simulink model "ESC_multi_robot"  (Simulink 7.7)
settings: Solver=ode3  StartTime=starttime  StopTime=stoptime  FixedStep=stepsize  RelTol=1e-3
PreLoadFcn:
  | load ESC_GUI_params_multi
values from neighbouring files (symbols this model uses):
  Kd = 60    [sim_run_multi.m]    (also in sim_run_uni.m)
  Kp = 3000    [sim_run_multi.m]    (also in sim_run_uni.m)
  noise_max = value    [ESC_GUI_multi.m]    (also in ESC_GUI_uni.m; sim_run_multi.m = 0.01; sim_run_uni.m = 0.2)
  switch_noise = 1    [ESC_GUI_multi.m]    (also in ESC_GUI_uni.m; sim_run_multi.m; sim_run_uni.m)
  switch_optimizer = method_no+1    [ESC_GUI_multi.m]    (also in ESC_GUI_uni.m = method_no; sim_run_multi.m = 4; sim_run_uni.m = 1)
  x0 = [0;0]    [sim_run_multi.m]    (also in sim_run_uni.m = 0)
undefined symbols (not defined in the file or in its folder): approx, nn, perturb
libraries: roblocks x8, simulink x1, commnoisgen2 x1

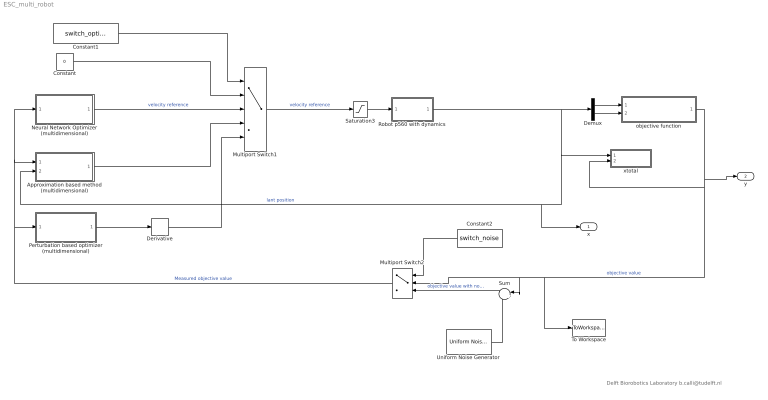
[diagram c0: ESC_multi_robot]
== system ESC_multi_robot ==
  note: Delft Biorobotics Laboratory b.calli@tudelft.nl
  Approximation based method (multidimensional) : Subsystem  mask{K_grad=approx.K_grad, sampling=approx.sampling, data_size=approx.data_size, vel_init=approx.vel_init, lpf_constant=approx.filter_constant}
      mask prompts: K_grad "Gain"; data_size "Data size"; vel_init "Initial velocity"; lpf_constant "Low pass filter constant"
  Constant : Constant  Value=0
  Constant1 : Constant  Value=switch_optimizer
  Constant2 : Constant  Value=switch_noise
  Demux : Demux  Outputs=2
  Derivative : Derivative
  Multiport Switch1 : MultiPortSwitch  Inputs=4  zeroidx=off
  Multiport Switch2 : MultiPortSwitch  Inputs=2  zeroidx=off
  Neural Network Optimizer (multidimensional) : Subsystem  mask{M=nn.M, A=nn.A, B=nn.B, ddelta1=nn.ddelta1, ddelta2=nn.ddelta2, ddelta3=nn.ddelta3, delta=nn.delta, mpd_init=nn.mpd_init}
      mask prompts: ddelta1 "Direction 1 delta"; ddelta2 "Direction 2 delta"; ddelta3 "Direction 3 delta"; mpd_init "Minimum Peak Detector initial value"
  Perturbation based optimizer (multidimensional) : Subsystem  mask{corr_gain=perturb.corr_gain, low_pass_pole=perturb.low_pass_pole, high_pass_pole=perturb.high_pass_pole, sine_amp=perturb.sine_amp, sine_freq=perturb.sine_freq, sine_phase=perturb.sine_phase, comp_zero=perturb.comp_zero, comp_pole=perturb.comp_pole}
      mask prompts: corr_gain "Correction gain"; low_pass_pole "Low Pass Filter pole"; high_pass_pole "High Pass Filter pole"; sine_amp "Sinus amplitude"; sine_freq "Sinus frequency"; sine_phase "Sinus phase"; comp_zero "Compensator zero"; comp_pole "Compensator pole"
  Robot p560 with dynamics : Subsystem
  Saturation3 : Saturate  UpperLimit=1  LowerLimit=-1
  Sum : Sum  Inputs=|++
  To Workspace : ToWorkspace  VariableName=y  SampleTime=-1  SaveFormat=Structure With Time
  Uniform Noise Generator : commnoisgen2/Uniform Noise Generator  SystemSampleTime=-1  low=-noise_max  up=noise_max  seed=31  Ts=0.001  frameBased=off  sampPerFrame=1  orient=off  outDataType=double
  objective function : Stateflow chart  TreatAsAtomicUnit=on
  xtotal : Subsystem
  x : Outport
  y : Outport  Port=2
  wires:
  Robot p560 with dynamics/1(x) -> xtotal/1(x), Approximation based method (multidimensional)/2(x), x/1, Demux/1  "lant position"
  Neural Network Optimizer (multidimensional)/1(xdot_ref) -> Multiport Switch1/3  "velocity reference"
  Constant/1 -> Multiport Switch1/2
  Constant1/1 -> Multiport Switch1/1
  objective function/1(y) -> Multiport Switch2/2, Sum/1, To Workspace/1, xtotal/2(y), y/1  "objective value"
  Uniform Noise Generator/1 -> Sum/2
  Sum/1 -> Multiport Switch2/3  "objective value with noise"
  Constant2/1 -> Multiport Switch2/1
  Approximation based method (multidimensional)/1(xdot_ref) -> Multiport Switch1/4
  Multiport Switch1/1 -> Saturation3/1  "velocity reference"
  Demux/1 -> objective function/1(x1)
  Perturbation based optimizer (multidimensional)/1(xref) -> Derivative/1
  Derivative/1 -> Multiport Switch1/5
  Multiport Switch2/1 -> Approximation based method (multidimensional)/1(y), Neural Network Optimizer (multidimensional)/1(y), Perturbation based optimizer (multidimensional)/1(y)  "Measured objective value"
  Demux/2 -> objective function/2(x2)
  Saturation3/1 -> Robot p560 with dynamics/1(xref)

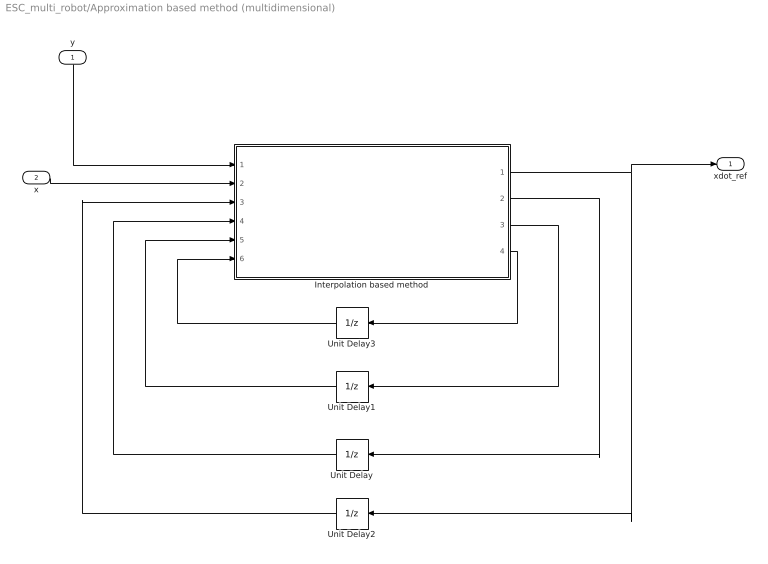
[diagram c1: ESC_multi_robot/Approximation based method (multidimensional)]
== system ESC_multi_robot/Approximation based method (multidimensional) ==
  y : Inport
  x : Inport  Port=2
  Interpolation based method : Stateflow chart  TreatAsAtomicUnit=on
  Unit Delay : UnitDelay  X0=[zeros(1,data_size);zeros(1,data_size)]  SampleTime=-1
  Unit Delay1 : UnitDelay  X0=zeros(1,data_size)  SampleTime=-1
  Unit Delay2 : UnitDelay  X0=[0;0]  SampleTime=-1
  Unit Delay3 : UnitDelay  SampleTime=-1
  xdot_ref : Outport
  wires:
  Unit Delay/1 -> Interpolation based method/4(x_data)
  Unit Delay1/1 -> Interpolation based method/5(y_data)
  y/1 -> Interpolation based method/1(y_data_in)
  x/1 -> Interpolation based method/2(x_data_in)
  Unit Delay2/1 -> Interpolation based method/3(xdot_ref_in)
  Unit Delay3/1 -> Interpolation based method/6(sample)
  Interpolation based method/4(sample_out) -> Unit Delay3/1
  Interpolation based method/3(y_data_out) -> Unit Delay1/1
  Interpolation based method/2(x_data_out) -> Unit Delay/1
  Interpolation based method/1(xdot_ref) -> Unit Delay2/1, xdot_ref/1

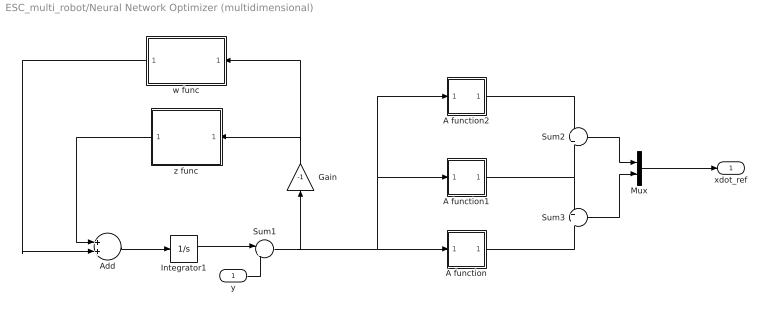
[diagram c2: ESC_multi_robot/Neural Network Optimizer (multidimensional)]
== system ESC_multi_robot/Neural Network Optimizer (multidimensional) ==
  y : Inport
  A function : Subsystem
  A function1 : Subsystem
  A function2 : Subsystem
  Add : Sum
  Gain : Gain  Gain=-1
  Integrator1 : Integrator  InitialCondition=mpd_init
  Mux : Mux  Inputs=2
  Sum1 : Sum  Inputs=|+-
  Sum2 : Sum  Inputs=+|+
  Sum3 : Sum  Inputs=+|+
  w func : Subsystem
  z func : Subsystem
  xdot_ref : Outport
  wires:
  Sum1/1 -> Gain/1, A function/1(e), A function1/1(e), A function2/1(e)
  Gain/1 -> w func/1(e_minus), z func/1(e_minus)
  w func/1(w) -> Add/2
  z func/1(z) -> Add/1
  Add/1 -> Integrator1/1
  Integrator1/1 -> Sum1/1
  A function2/1(xdot) -> Sum2/1
  A function1/1(xdot) -> Sum2/2, Sum3/1
  A function/1(xdot) -> Sum3/2
  Sum2/1 -> Mux/1
  Sum3/1 -> Mux/2
  Mux/1 -> xdot_ref/1
  y/1 -> Sum1/2

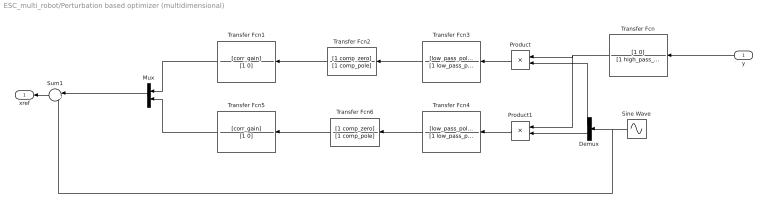
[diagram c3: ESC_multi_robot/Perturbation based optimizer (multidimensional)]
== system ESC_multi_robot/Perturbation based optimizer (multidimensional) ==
  y : Inport
  Demux : Demux  Outputs=2
  Mux : Mux  Inputs=2
  Product : Product  Multiplication=Matrix(*)
  Product1 : Product  Multiplication=Matrix(*)
  Sine Wave : Sin  Amplitude=[sine_amp sine_amp]  Frequency=[sine_freq sine_freq]  Phase=[0 sine_phase]  SampleTime=0
  Sum1 : Sum  Inputs=|++
  Transfer Fcn : TransferFcn  Numerator=[1 0]  Denominator=[1 high_pass_pole]
  Transfer Fcn1 : TransferFcn  Numerator=[corr_gain]  Denominator=[1 0]
  Transfer Fcn2 : TransferFcn  Numerator=[1 comp_zero]  Denominator=[1 comp_pole]
  Transfer Fcn3 : TransferFcn  Numerator=[low_pass_pole]  Denominator=[1 low_pass_pole]
  Transfer Fcn4 : TransferFcn  Numerator=[low_pass_pole]  Denominator=[1 low_pass_pole]
  Transfer Fcn5 : TransferFcn  Numerator=[corr_gain]  Denominator=[1 0]
  Transfer Fcn6 : TransferFcn  Numerator=[1 comp_zero]  Denominator=[1 comp_pole]
  xref : Outport
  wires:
  y/1 -> Transfer Fcn/1
  Sum1/1 -> xref/1
  Transfer Fcn/1 -> Product/1, Product1/1
  Sine Wave/1 -> Demux/1, Sum1/2
  Demux/1 -> Product/2
  Demux/2 -> Product1/2
  Product/1 -> Transfer Fcn3/1
  Product1/1 -> Transfer Fcn4/1
  Transfer Fcn3/1 -> Transfer Fcn2/1
  Transfer Fcn4/1 -> Transfer Fcn6/1
  Transfer Fcn1/1 -> Mux/1
  Transfer Fcn5/1 -> Mux/2
  Mux/1 -> Sum1/1
  Transfer Fcn2/1 -> Transfer Fcn1/1
  Transfer Fcn6/1 -> Transfer Fcn5/1

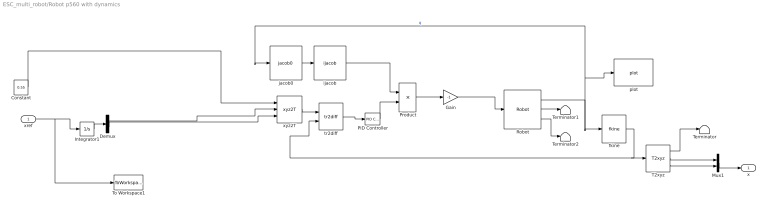
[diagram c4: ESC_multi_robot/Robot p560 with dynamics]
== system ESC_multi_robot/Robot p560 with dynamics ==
  xref : Inport
  Constant : Constant  Value=0.55
  Demux : Demux  Outputs=2
  Gain : Gain  Gain=-1
  Integrator1 : Integrator  InitialCondition=x0
  Mux1 : Mux  Inputs=2
  PID Controller : simulink/Continuous/PID Controller  SystemSampleTime=-1  Controller=PID  TimeDomain=Continuous-time  SampleTime=1  IntegratorMethod=Forward Euler  FilterMethod=Forward Euler  Form=Parallel  P=[Kp Kp Kp Kp Kp Kp]  I=[0 0 0 0 0 0]  D=[Kd Kd Kd Kd Kd Kd]  N=100  InitialConditionSource=internal  InitialConditionForIntegrator=0  InitialConditionForFilter=0  ExternalReset=none  LimitOutput=off  UpperSaturationLimit=inf  LowerSaturationLimit=-inf  LinearizeAsGain=off  AntiWindupMode=none  Kb=1  TrackingMode=off  Kt=1  PParamMin=[]  PParamMax=[]  IParamMin=[]  IParamMax=[]  DParamMin=[]  DParamMax=[]  NParamMin=[]  NParamMax=[]  KbParamMin=[]  KbParamMax=[]  KtParamMin=[]  KtParamMax=[]  POutMin=[]  POutMax=[]  IOutMin=[]  IOutMax=[]  DOutMin=[]  DOutMax=[]  NOutMin=[]  NOutMax=[]  KbOutMin=[]  KbOutMax=[]  KtOutMin=[]  KtOutMax=[]  IntegratorOutMin=[]  IntegratorOutMax=[]  FilterOutMin=[]  FilterOutMax=[]  SumOutMin=[]  SumOutMax=[]  SumI1OutMin=[]  SumI1OutMax=[]  SumI2OutMin=[]  SumI2OutMax=[]  SumI3OutMin=[]  SumI3OutMax=[]  SumDOutMin=[]  SumDOutMax=[]  SaturationOutMin=[]  SaturationOutMax=[]  IntegratorContinuousStateAttributes=''  IntegratorStateMustResolveToSignalObject=off  IntegratorRTWStateStorageClass=Auto  FilterContinuousStateAttributes=''  FilterStateMustResolveToSignalObject=off  FilterRTWStateStorageClass=Auto
  Product : Product  Multiplication=Matrix(*)
  Robot : roblocks/Robot  SystemSampleTime=-1  robot=p560  q0="[0.2763    0.9125    2.9359         0    2.4348   -0.2763]"
  T2xyz : roblocks/T2xyz  SystemSampleTime=-1
  Terminator : Terminator
  Terminator1 : Terminator
  Terminator2 : Terminator
  To Workspace1 : ToWorkspace  VariableName=u_out  SampleTime=-1  SaveFormat=Structure With Time
  fkine : roblocks/fkine  SystemSampleTime=-1  robot=p560
  ijacob : roblocks/ijacob  SystemSampleTime=-1
  jacob0 : roblocks/jacob0   SystemSampleTime=-1  robot=p560
  plot : roblocks/plot  SystemSampleTime=-1  robot=p560
  tr2diff : roblocks/tr2diff  SystemSampleTime=-1  robot=robot
  xyz2T : roblocks/xyz2T  SystemSampleTime=-1
  x : Outport
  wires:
  xref/1 -> Integrator1/1, To Workspace1/1
  Integrator1/1 -> Demux/1
  Robot/1 -> fkine/1, jacob0/1, plot/1  "q"
  tr2diff/1 -> PID Controller/1
  xyz2T/1 -> tr2diff/1
  fkine/1 -> T2xyz/1, tr2diff/2
  jacob0/1 -> ijacob/1
  ijacob/1 -> Product/1
  Product/1 -> Gain/1
  Gain/1 -> Robot/1
  PID Controller/1 -> Product/2
  Robot/2 -> Terminator1/1
  Robot/3 -> Terminator2/1
  Demux/1 -> xyz2T/2
  Constant/1 -> xyz2T/1
  Demux/2 -> xyz2T/3
  Mux1/1 -> x/1
  T2xyz/2 -> Mux1/1
  T2xyz/3 -> Mux1/2
  T2xyz/1 -> Terminator/1

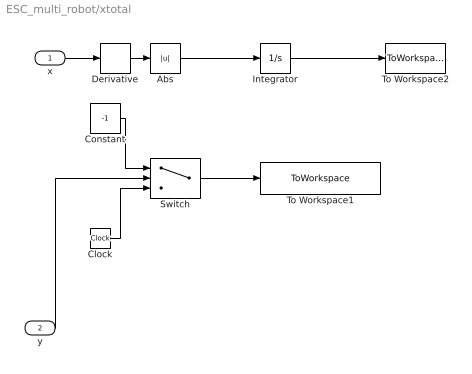
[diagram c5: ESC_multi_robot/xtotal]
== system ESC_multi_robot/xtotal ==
  x : Inport
  y : Inport  Port=2
  Abs : Abs
  Clock : Clock
  Constant : Constant  Value=-1
  Derivative : Derivative
  Integrator : Integrator
  Switch : Switch  Threshold=1.05
  To Workspace1 : ToWorkspace  VariableName=peak_time_detector  SampleTime=-1  SaveFormat=Array
  To Workspace2 : ToWorkspace  VariableName=x_total  SampleTime=-1  SaveFormat=Array
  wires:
  y/1 -> Switch/2
  Clock/1 -> Switch/3
  Switch/1 -> To Workspace1/1
  Constant/1 -> Switch/1
  x/1 -> Derivative/1
  Integrator/1 -> To Workspace2/1
  Abs/1 -> Integrator/1
  Derivative/1 -> Abs/1

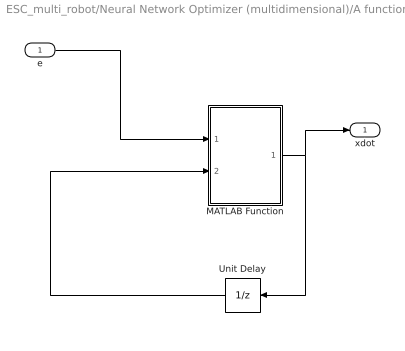
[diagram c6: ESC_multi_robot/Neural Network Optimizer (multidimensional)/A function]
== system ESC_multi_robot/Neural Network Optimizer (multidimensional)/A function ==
  e : Inport
  MATLAB Function : Stateflow chart  TreatAsAtomicUnit=on
  Unit Delay : UnitDelay  X0=A  SampleTime=-1
  xdot : Outport
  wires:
  Unit Delay/1 -> MATLAB Function/2(state_pre)
  MATLAB Function/1(xdot) -> xdot/1, Unit Delay/1
  e/1 -> MATLAB Function/1(e)

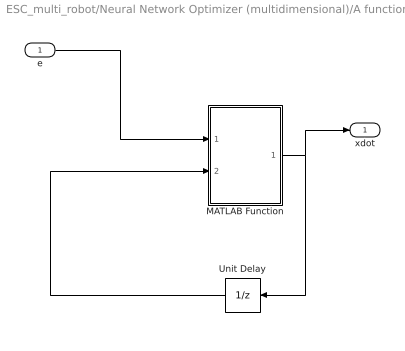
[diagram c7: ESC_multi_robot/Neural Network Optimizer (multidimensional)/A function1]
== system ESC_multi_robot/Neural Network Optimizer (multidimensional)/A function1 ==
  e : Inport
  MATLAB Function : Stateflow chart  TreatAsAtomicUnit=on
  Unit Delay : UnitDelay  SampleTime=-1
  xdot : Outport
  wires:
  e/1 -> MATLAB Function/1(e)
  MATLAB Function/1(xdot) -> Unit Delay/1, xdot/1
  Unit Delay/1 -> MATLAB Function/2(state_pre)

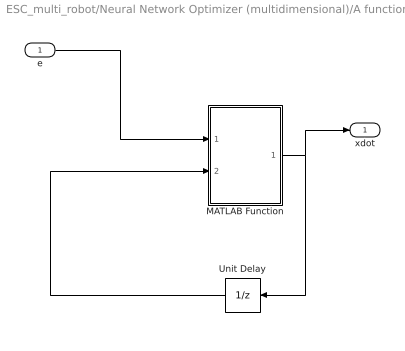
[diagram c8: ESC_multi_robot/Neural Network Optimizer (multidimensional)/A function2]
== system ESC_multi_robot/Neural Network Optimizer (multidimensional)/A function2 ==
  e : Inport
  MATLAB Function : Stateflow chart  TreatAsAtomicUnit=on
  Unit Delay : UnitDelay  SampleTime=-1
  xdot : Outport
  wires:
  Unit Delay/1 -> MATLAB Function/2(state_pre)
  MATLAB Function/1(xdot) -> xdot/1, Unit Delay/1
  e/1 -> MATLAB Function/1(e)

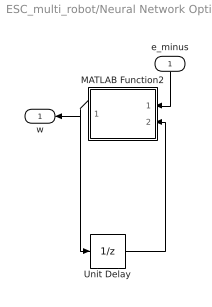
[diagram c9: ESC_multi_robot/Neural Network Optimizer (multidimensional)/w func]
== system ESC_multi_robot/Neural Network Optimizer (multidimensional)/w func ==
  e_minus : Inport
  MATLAB Function2 : Stateflow chart  TreatAsAtomicUnit=on
  Unit Delay : UnitDelay  SampleTime=-1
  w : Outport
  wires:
  e_minus/1 -> MATLAB Function2/1(e_minus)
  MATLAB Function2/1(w) -> w/1, Unit Delay/1
  Unit Delay/1 -> MATLAB Function2/2(state_pre)

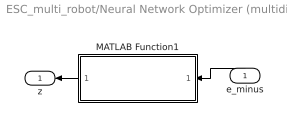
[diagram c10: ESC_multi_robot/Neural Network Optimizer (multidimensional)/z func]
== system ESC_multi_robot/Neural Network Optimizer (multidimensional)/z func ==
  e_minus : Inport
  MATLAB Function1 : Stateflow chart  TreatAsAtomicUnit=on
  z : Outport
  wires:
  e_minus/1 -> MATLAB Function1/1(e_minus)
  MATLAB Function1/1(z) -> z/1

== matlab function Approximation based method
(multidimensional)/Interpolation based
method ==
function [xdot_ref,x_data_out,y_data_out, sample_out] = interpolation_based_method(y_data_in, x_data_in, xdot_ref_in, x_data, y_data,K_grad, sample, sampling, data_size, vel_init, lpf_constant)
%#codegen
if(mod(sample,sampling) == 0 )
    sample_out = sample+1;
    x1_data = x_data(1,:);
    x2_data = x_data(2,:);
    x1_data = circshift(x1_data,[0,1]);
    x2_data = circshift(x2_data,[0,1]);
    y_data = circshift(y_data,1);
    x1_data(1) = x_data_in(1,1);
    x2_data(1) = x_data_in(2,1);
    y_data(1) = y_data_in;
    
    V = zeros(data_size,4);
    
    for i=1:data_size
        V(i,:) = [x1_data(i)*x2_data(i) x1_data(i) x2_data(i) 1];
    end

    c = pinv(V)*y_data;
    x = [x1_data(1);x2_data(1)];
    grad_val = [c(1)*x(2)+c(2);
                c(1)*x(1)+c(3)];
    %grad_val = grad_val./norm(grad_val,1);

    if (sample<sampling*data_size)
        xdot_ref = [vel_init;vel_init];
    else
        xdot_ref = -K_grad*grad_val;
        
        if (xdot_ref(1)~=xdot_ref(1) || xdot_ref(2)~=xdot_ref(2))
            xdot_ref = [0;0];
        end
    end

    if(xdot_ref(1)==vel_init && xdot_ref(2)==vel_init)
    else
        xdot_ref(1) = lpf_constant * xdot_ref(1) + ( 1.0 - lpf_constant ) * xdot_ref_in(1);
        xdot_ref(2) = lpf_constant * xdot_ref(2) + ( 1.0 - lpf_constant ) * xdot_ref_in(2);
    end
    
    x_data_out = [x1_data; x2_data];
    y_data_out = y_data;
else
    sample_out = sample+1;
    x_data_out = x_data;
    y_data_out = y_data;
    xdot_ref = xdot_ref_in;
end

== matlab function Neural Network Optimizer
(multidimensional)/A function/MATLAB Function ==
function xdot = fnc(e,state_pre,A,ddelta1)
%#codegen

if( e<-ddelta1 )
    xdot = -A;
elseif(e>ddelta1)
    xdot = A;
else
    xdot = state_pre;
end

end

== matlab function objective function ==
function y = objective_function(x1,x2)
%#codegen

y= obj_func_multi(x1,x2);

== matlab function Neural Network Optimizer
(multidimensional)/A function1/MATLAB Function ==
function xdot = fnc1(e,state_pre,A,ddelta2)
%#codegen

if( e<-ddelta2 )
    xdot = 0;
elseif(e>ddelta2)
    xdot = A;
else
    xdot = state_pre;
end

end

== matlab function Neural Network Optimizer
(multidimensional)/A function2/MATLAB Function ==
function xdot = fnc3(e,state_pre,A,ddelta3)
%#codegen

if( e<-ddelta3 )
    xdot = -2*A;
elseif(e>ddelta3)
    xdot = 0;
else
    xdot = state_pre;
end

end

== matlab function Neural Network Optimizer
(multidimensional)/w func/MATLAB Function2 ==
function w = wfunc(e_minus,state_pre,B,delta)
%#codegen
if(e_minus<-delta)
    w = 0;
elseif (e_minus>delta)
    w = B;
else
    w = state_pre;
end
end

== matlab function Neural Network Optimizer
(multidimensional)/z func/MATLAB Function1 ==
function z = zfunc(e_minus,M)
%#codegen
if(e_minus>0)
    z = 0;
else
    z = -M;
end
end
